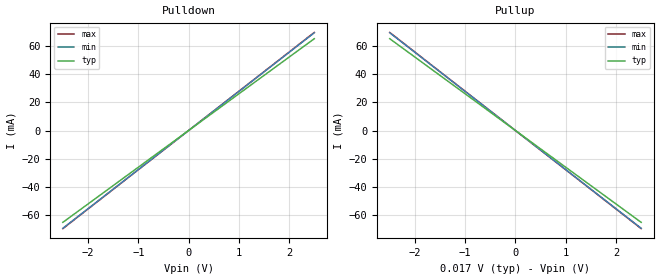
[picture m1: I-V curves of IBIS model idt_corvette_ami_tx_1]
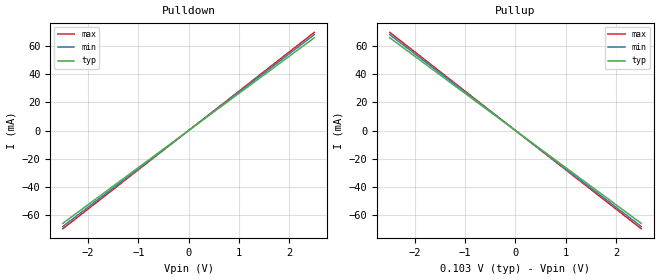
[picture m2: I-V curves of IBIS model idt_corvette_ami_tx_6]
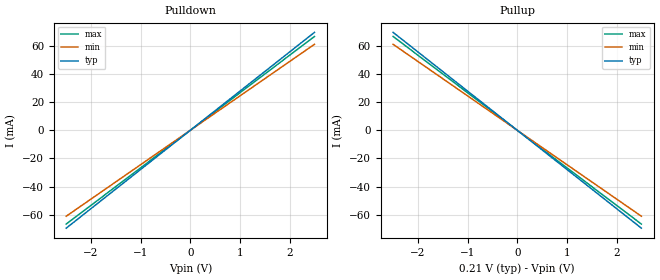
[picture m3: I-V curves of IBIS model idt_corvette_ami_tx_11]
|   IDT Corvette Transceiver IBIS-AMI Models
[IBIS Ver]   5.1
[Disclaimer]
   This is a preliminary model and is subject to change.
   Integrated Device Technology, Inc. ("IDT") hereby grants the
   user of this IBIS model a non-exclusive, nontransferable
   license to use this IBIS model under the following terms. The
   user is granted this license only to use the IBIS model and is
   not granted rights to sell, copy (except as needed to run the
   IBIS model), rent, lease or sub-license the IBIS model in
   whole or in part, or in modified form to anyone. The User may
   modify the IBIS model to suit its specific applications, but
   rights to derivative works and such modifications shall belong
   to IDT. This IBIS model is provided on an AS IS" basis and IDT
   makes absolutely no warranty with respect to the information
   contained herein. IDT DISCLAIMS AND CUSTOMER WAIVES ALL
   WARRANTIES, EXPRESS AND IMPLIED, INCLUDING WARRANTIES OF
   MERCHANTABILITY AND FITNESS FOR A PARTICULAR PURPOSE. THE
   ENTIRE RISK AS TO QUALITY AND PERFORMANCE IS WITH THE USER
   ACCORDINGLY, IN NO EVENT SHALL IDT BE LIABLE FOR ANY DIRECT OR
   INDIRECT DAMAGES, WHETHER IN CONTRACT OR TORT, INCLUDING ANY
   LOST PROFITS OR OTHER INCIDENTAL, CONSEQUENTIAL, EXEMPLARY, OR
   PUNITIVE DAMAGES ARISING OUT OF THE USE OR APPLICATION OF THE
   IBIS model. Further, IDT reserves the right to make changes
   without notice to any product herein to improve reliability,
   function, or design. IDT does not convey any license under
   patent rights or any other intellectual property rights,
   including those of third parties. IDT is not obligated to
   provide maintenance or support for the licensed IBIS model.
[File Name]  idt_corvette.ibs
[Date]   February 6, 2014
[File Rev]   5.1
[Source]   Integrated Device Techology, Inc. (IDT)
[Notes]
   Revision 1.0 -- 3/23/2010 : Initial release
   Revision 1.1 -- 4/23/2010 : Revised model header
   Revision 3.0 -- 9/02/2011 : Updated TX Models based on lab data.
   - Passes ibischk v5.0.6 with 0 errors and 34 warnings. All warnings
   are due to Voltage Range values that are not in Typ-Min-Max order.
   Since the Voltage Range values are correct for the Typ-Min-Max
   process corners, these warnings can be ignored.
   Revision 3.1 -- 9/02/2011 : made TX AMP 31 default model to match AM
   Revision 4.0  -- 9/20/2011: Model updated to match LAB data/
   84 warnings due to Type not between Min/Max
   for voltage. These can be ignored
   Revision 5.0  -- 2/4/2014: Model updated to support 64b Linux and Windows
   Revision 5.1  -- 2/6/2014: Updated file and syntax to IBIS version 5.1
   File passes IBISCHK v5.1.4 with 0 Errors and 28 Warnings.
   All warnings are due to typ voltage value not being between
   min and max. These warnings are expected (the values are correct)
   and can be ignored.
[Copyright]  Copyright 2014, IDT, All Rights Reserved.
|   COMPONENT: corvette_serdes R5.1
[Component] corvette_serdes
[Manufacturer]  IDT
[Package]
R_pkg   0.001m  NA NA
L_pkg   0.001nH NA NA
C_pkg   0.001pF NA NA
[Pin] signal_name   model_name   R_pin L_pin C_pin
1   corvette_rx_p   idt_corvette_ami_rx   NA   NA   NA
2   corvette_rx_n   idt_corvette_ami_rx   NA   NA   NA
5   corvette_tx_p   idt_corvette_ami_tx   NA   NA   NA
6   corvette_tx_n   idt_corvette_ami_tx   NA   NA   NA
[Diff Pin] inv_pin  vdiff tdelay_typ tdelay_min tdelay_max
1 2 0.025 na na na
5 6 0.025 na na na
[Model Selector] idt_corvette_ami_tx
idt_corvette_ami_tx_31   TX Amp Setting 31 (Default setting)
idt_corvette_ami_tx_0   TX Amp Setting 0
idt_corvette_ami_tx_1   TX Amp Setting 1
idt_corvette_ami_tx_2   TX Amp Setting 2
idt_corvette_ami_tx_3   TX Amp Setting 3
idt_corvette_ami_tx_4   TX Amp Setting 4
idt_corvette_ami_tx_5   TX Amp Setting 5
idt_corvette_ami_tx_6   TX Amp Setting 6
idt_corvette_ami_tx_7   TX Amp Setting 7
idt_corvette_ami_tx_8   TX Amp Setting 8
idt_corvette_ami_tx_9   TX Amp Setting 9
idt_corvette_ami_tx_10   TX Amp Setting 10
idt_corvette_ami_tx_11   TX Amp Setting 11
idt_corvette_ami_tx_12   TX Amp Setting 12
idt_corvette_ami_tx_13   TX Amp Setting 13
idt_corvette_ami_tx_14   TX Amp Setting 14
idt_corvette_ami_tx_15   TX Amp Setting 15
idt_corvette_ami_tx_16   TX Amp Setting 16
idt_corvette_ami_tx_17   TX Amp Setting 17
idt_corvette_ami_tx_18   TX Amp Setting 18
idt_corvette_ami_tx_19   TX Amp Setting 19
idt_corvette_ami_tx_20   TX Amp Setting 20
idt_corvette_ami_tx_21   TX Amp Setting 21
idt_corvette_ami_tx_22   TX Amp Setting 22
idt_corvette_ami_tx_23   TX Amp Setting 23
idt_corvette_ami_tx_24   TX Amp Setting 24
idt_corvette_ami_tx_25   TX Amp Setting 25
idt_corvette_ami_tx_26   TX Amp Setting 26
idt_corvette_ami_tx_27   TX Amp Setting 27
idt_corvette_ami_tx_28   TX Amp Setting 28
idt_corvette_ami_tx_29   TX Amp Setting 29
idt_corvette_ami_tx_30   TX Amp Setting 30
|||idt_corvette_ami_tx_31   TX Amp Setting 31 ||Defined as default above
idt_corvette_ami_tx_32   TX Amp Setting 32
idt_corvette_ami_tx_33   TX Amp Setting 33
idt_corvette_ami_tx_34   TX Amp Setting 34
idt_corvette_ami_tx_35   TX Amp Setting 35
idt_corvette_ami_tx_36   TX Amp Setting 36
idt_corvette_ami_tx_37   TX Amp Setting 37
idt_corvette_ami_tx_38   TX Amp Setting 38
idt_corvette_ami_tx_39   TX Amp Setting 39
idt_corvette_ami_tx_40   TX Amp Setting 40
idt_corvette_ami_tx_41   TX Amp Setting 41
idt_corvette_ami_tx_42   TX Amp Setting 42
idt_corvette_ami_tx_43   TX Amp Setting 43
idt_corvette_ami_tx_44   TX Amp Setting 44
idt_corvette_ami_tx_45   TX Amp Setting 45
idt_corvette_ami_tx_46   TX Amp Setting 46
idt_corvette_ami_tx_47   TX Amp Setting 47
idt_corvette_ami_tx_48   TX Amp Setting 48
idt_corvette_ami_tx_49   TX Amp Setting 49
idt_corvette_ami_tx_50   TX Amp Setting 50
idt_corvette_ami_tx_51   TX Amp Setting 51
idt_corvette_ami_tx_52   TX Amp Setting 52
idt_corvette_ami_tx_53   TX Amp Setting 53
idt_corvette_ami_tx_54   TX Amp Setting 54
idt_corvette_ami_tx_55   TX Amp Setting 55
idt_corvette_ami_tx_56   TX Amp Setting 56
idt_corvette_ami_tx_57   TX Amp Setting 57
idt_corvette_ami_tx_58   TX Amp Setting 58
idt_corvette_ami_tx_59   TX Amp Setting 59
idt_corvette_ami_tx_60   TX Amp Setting 60
idt_corvette_ami_tx_61   TX Amp Setting 61
idt_corvette_ami_tx_62   TX Amp Setting 62
idt_corvette_ami_tx_63   TX Amp Setting 63
| Models and submodels in the file (65): idt_corvette_ami_tx_0 (Output), idt_corvette_ami_tx_1 (Output), idt_corvette_ami_tx_2 (Output), idt_corvette_ami_tx_3 (Output), idt_corvette_ami_tx_4 (Output), idt_corvette_ami_tx_5 (Output), idt_corvette_ami_tx_6 (Output), idt_corvette_ami_tx_7 (Output), idt_corvette_ami_tx_8 (Output), idt_corvette_ami_tx_9 (Output), idt_corvette_ami_tx_10 (Output), idt_corvette_ami_tx_11 (Output), idt_corvette_ami_tx_12 (Output), idt_corvette_ami_tx_13 (Output), idt_corvette_ami_tx_14 (Output), idt_corvette_ami_tx_15 (Output), idt_corvette_ami_tx_16 (Output), idt_corvette_ami_tx_17 (Output), idt_corvette_ami_tx_18 (Output), idt_corvette_ami_tx_19 (Output), idt_corvette_ami_tx_20 (Output), idt_corvette_ami_tx_21 (Output), idt_corvette_ami_tx_22 (Output), idt_corvette_ami_tx_23 (Output), idt_corvette_ami_tx_24 (Output), idt_corvette_ami_tx_25 (Output), idt_corvette_ami_tx_26 (Output), idt_corvette_ami_tx_27 (Output), idt_corvette_ami_tx_28 (Output), idt_corvette_ami_tx_29 (Output), idt_corvette_ami_tx_30 (Output), idt_corvette_ami_tx_31 (Output), idt_corvette_ami_tx_32 (Output), idt_corvette_ami_tx_33 (Output), idt_corvette_ami_tx_34 (Output), idt_corvette_ami_tx_35 (Output), idt_corvette_ami_tx_36 (Output), idt_corvette_ami_tx_37 (Output), idt_corvette_ami_tx_38 (Output), idt_corvette_ami_tx_39 (Output), idt_corvette_ami_tx_40 (Output), idt_corvette_ami_tx_41 (Output), idt_corvette_ami_tx_42 (Output), idt_corvette_ami_tx_43 (Output), idt_corvette_ami_tx_44 (Output), idt_corvette_ami_tx_45 (Output), idt_corvette_ami_tx_46 (Output), idt_corvette_ami_tx_47 (Output), idt_corvette_ami_tx_48 (Output), idt_corvette_ami_tx_49 (Output), idt_corvette_ami_tx_50 (Output), idt_corvette_ami_tx_51 (Output), idt_corvette_ami_tx_52 (Output), idt_corvette_ami_tx_53 (Output), idt_corvette_ami_tx_54 (Output), idt_corvette_ami_tx_55 (Output), idt_corvette_ami_tx_56 (Output), idt_corvette_ami_tx_57 (Output), idt_corvette_ami_tx_58 (Output), idt_corvette_ami_tx_59 (Output), idt_corvette_ami_tx_60 (Output), idt_corvette_ami_tx_61 (Output), idt_corvette_ami_tx_62 (Output), idt_corvette_ami_tx_63 (Output), idt_corvette_ami_rx (Input)
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|   model   idt_corvette_ami_tx_1
[Model] idt_corvette_ami_tx_1
Model_type Output
C_comp 400f 400f 400f
Cref = 0
[Model Spec]
Vmeas 0. 0. 0.
Vref 0. 0. 0.
[Temperature Range]  25 100 0
[Voltage Range] .0171 .0164 .0157
[Algorithmic Model]
Executable Windows_VisualStudio5_32 idt_corvette_tx.dll   idt_corvette_tx.ami
Executable Windows_ver_64   idt_corvette_tx_64.dll   idt_corvette_tx.ami
Executable Linux_gcc4.1.2_32   idt_corvette_tx.linux.so   idt_corvette_tx.ami
Executable Linux_gcc3.2.3_64   idt_corvette_tx_64.linux.so idt_corvette_tx.ami
[End Algorithmic Model]
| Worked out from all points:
|   slope of the pulldown table from 0 to 0.003 V, typ, clamps not added: 38.5 ohm
|   slope of the pullup table from 0 to 0.003 V, typ, clamps not added: 38.5 ohm
[Pulldown]
-2.5V     -64.98mA   -69.17mA   -69.44mA
0V        0A         0A         0A
2.5V      64.98mA    69.17mA    69.44mA
[Pullup]
-2.5V     64.98mA    69.17mA    69.44mA
0V        0A         0A         0A
2.5V      -64.98mA   -69.17mA   -69.44mA
[Ramp]
dV/dt_r .00581/21.544p .00572/20.24p .00548/20.16p
dV/dt_f .00581/21.544p .00572/20.24p .00548/20.16p
|   model   idt_corvette_ami_tx_6
[Model] idt_corvette_ami_tx_6
Model_type Output
C_comp 400f 400f 400f
Cref = 0
[Model Spec]
Vmeas 0. 0. 0.
Vref 0. 0. 0.
[Temperature Range]  25 100 0
[Voltage Range] .103 .0986 .0943
[Algorithmic Model]
Executable Windows_VisualStudio5_32 idt_corvette_tx.dll   idt_corvette_tx.ami
Executable Windows_ver_64   idt_corvette_tx_64.dll   idt_corvette_tx.ami
Executable Linux_gcc4.1.2_32   idt_corvette_tx.linux.so   idt_corvette_tx.ami
Executable Linux_gcc3.2.3_64   idt_corvette_tx_64.linux.so idt_corvette_tx.ami
[End Algorithmic Model]
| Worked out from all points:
|   slope of the pulldown table from 0 to 0.015 V, typ, clamps not added: 38.1 ohm
|   slope of the pullup table from 0 to 0.015 V, typ, clamps not added: 38.1 ohm
[Pulldown]
-2.5V     -65.65mA   -67.83mA   -69.44mA
0V        0A         0A         0A
2.5V      65.65mA    67.83mA    69.44mA
[Pullup]
-2.5V     65.65mA    67.83mA    69.44mA
0V        0A         0A         0A
2.5V      -65.65mA   -67.83mA   -69.44mA
[Ramp]
dV/dt_r .035/21.324p .0341/20.64p .0329/20.16p
dV/dt_f .035/21.324p .0341/20.64p .0329/20.16p
|   model   idt_corvette_ami_tx_11
[Model] idt_corvette_ami_tx_11
Model_type Output
C_comp 400f 400f 400f
Cref = 0
[Model Spec]
Vmeas 0. 0. 0.
Vref 0. 0. 0.
[Temperature Range]  25 100 0
[Voltage Range] .21 .21 .185
[Algorithmic Model]
Executable Windows_VisualStudio5_32 idt_corvette_tx.dll   idt_corvette_tx.ami
Executable Windows_ver_64   idt_corvette_tx_64.dll   idt_corvette_tx.ami
Executable Linux_gcc4.1.2_32   idt_corvette_tx.linux.so   idt_corvette_tx.ami
Executable Linux_gcc3.2.3_64   idt_corvette_tx_64.linux.so idt_corvette_tx.ami
[End Algorithmic Model]
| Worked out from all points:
|   slope of the pulldown table from 0 to 0.032 V, typ, clamps not added: 36 ohm
|   slope of the pullup table from 0 to 0.032 V, typ, clamps not added: 36 ohm
[Pulldown]
-2.5V     -69.44mA   -60.98mA   -66.53mA
0V        0A         0A         0A
2.5V      69.44mA    60.98mA    66.53mA
[Pullup]
-2.5V     69.44mA    60.98mA    66.53mA
0V        0A         0A         0A
2.5V      -69.44mA   -60.98mA   -66.53mA
[Ramp]
dV/dt_r .0733/20.16p .0692/22.96p .0634/21.042p
dV/dt_f .0733/20.16p .0692/22.96p .0634/21.042p
